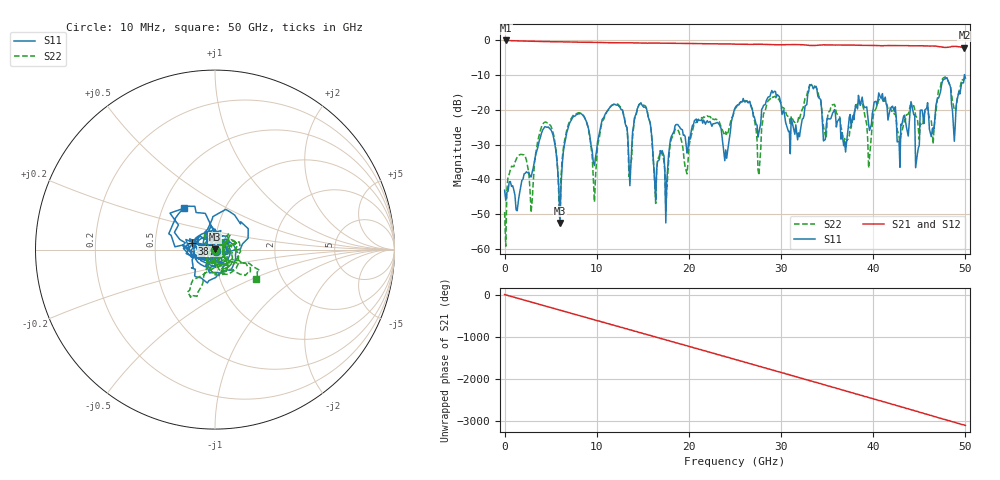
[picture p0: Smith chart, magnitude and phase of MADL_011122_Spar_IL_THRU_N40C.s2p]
#	HZ	S	DB	R	50
!Frequency	S11 (dB)	S11-Ang	S21 (dB)	S21-Ang	S12 (dB)	S12-Ang	S22 (dB)	S22-Ang
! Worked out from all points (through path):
!   401 points, 10 MHz to 50 GHz, reference 50 ohm
!   highest |S21| = 0.00 dB at 135 MHz (marker M1); lowest = -2.0 dB at 49.9 GHz (marker M2)
!   group delay of S21, straight-line fit = 172 ps
!   lowest |S11| = -52.5 dB at 6.01 GHz (marker M3), VSWR 1.00, Z = 50.1 + j0.221 ohm
!   |S11| at or under -10 dB: start of sweep to 49.89 GHz; 49.91837 GHz to end of sweep
!   |S22| runs from -59.2 to -10.5 dB; largest |S21 - S12| = 0.016
!   S11 on the Smith chart (normalised r, x): 10 MHz: 1.01, -0.01; 38.5 GHz: 0.77, +0.05; 50 GHz: 0.64, +0.32
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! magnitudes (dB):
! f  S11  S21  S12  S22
! 10 MHz  -43.1  0.0  0.0  -49.4
! 135 MHz  -46.0  0.0  0.0  -59.2
! 3.01 GHz  -37.9  -0.3  -0.3  -45.8
! 4.38 GHz  -24.8  -0.3  -0.3  -23.5
! 6.01 GHz  -52.5  -0.4  -0.4  -53.4
! 8.38 GHz  -21.2  -0.5  -0.5  -21.1
! 9.76 GHz  -36.0  -0.5  -0.5  -46.5
! 12 GHz  -18.4  -0.7  -0.7  -18.2
! 16.8 GHz  -34.3  -0.8  -0.8  -33.2
! 24 GHz  -31.5  -1.0  -1.0  -26.3
! 25.1 GHz  -19.0  -1.1  -1.1  -19.4
! 27.5 GHz  -27.8  -1.1  -1.1  -37.1
! 28.6 GHz  -16.3  -1.2  -1.2  -17.3
! 31.8 GHz  -28.6  -1.2  -1.2  -23.5
! 33.4 GHz  -13.1  -1.4  -1.5  -12.6
! 36.9 GHz  -29.1  -1.3  -1.3  -28.2
! 38.5 GHz  -17.6  -1.4  -1.4  -17.4
! 39.5 GHz  -24.1  -1.4  -1.4  -36.7
! 41.8 GHz  -20.1  -1.5  -1.5  -19.3
! 44.8 GHz  -32.5  -1.5  -1.5  -22.6
! 49.9 GHz  -9.8  -2.0  -2.1  -10.8
! 50 GHz  -10.8  -2.0  -2.0  -11.0
